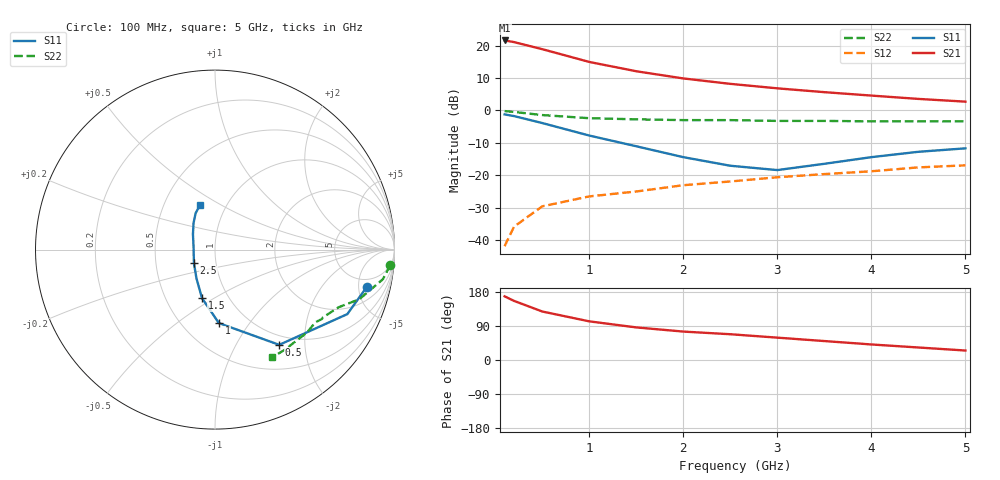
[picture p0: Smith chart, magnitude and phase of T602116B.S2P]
!AT-60211
!S-PARAMETERS at Vce=6V  Ic=5mA.  LAST UPDATED 07-21-92
# ghz s ma r 50
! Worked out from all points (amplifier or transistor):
!   12 points, 100 MHz to 5 GHz, reference 50 ohm
!   highest |S21| = 21.6 dB at 100 MHz (marker M1)
!   |S21| within 3 dB of that: start of sweep to 539.3 MHz
!   unconditionally stable (mu >= 1): 1.411 GHz to end of sweep
!   at 500 MHz: K = 0.50, MSG = 24.3 dB, |S12| = -29.6 dB
!   at 2.5 GHz: K = 1.22, MAG = 12.3 dB, |S12| = -21.9 dB
!   at 5 GHz: K = 1.23, MAG = 6.9 dB, |S12| = -17.0 dB
!   S11 on the Smith chart (normalised r, x): 100 MHz: 3.54, -6.14; 500 MHz: 0.85, -1.53; 1 GHz: 0.74, -0.73; 1.5 GHz: 0.75, -0.44; 2.5 GHz: 0.78, -0.12; 5 GHz: 0.75, +0.40
0.1  0.87 -14.0  12.09 168.0  0.008 80.0  0.98 -5.0
0.2  0.82 -26.0  11.41 156.0  0.016 80.0  0.95 -10.0
0.5  0.64 -56.0  8.87 128.0  0.033 59.0  0.85 -19.0
1  0.41 -87.0  5.63 102.0  0.047 54.0  0.76 -25.0
1.5  0.28 -105.0  4.04 86.0  0.056 54.0  0.73 -29.0
2  0.19 -123.0  3.13 75.0  0.07 56.0  0.71 -32.0
2.5  0.14 -147.0  2.58 68.0  0.08 60.0  0.71 -33.0
3  0.12 174.0  2.2 59.0  0.093 58.0  0.69 -36.0
3.5  0.15 145.0  1.92 50.0  0.104 58.0  0.69 -42.0
4  0.19 129.0  1.7 41.0  0.115 56.0  0.68 -49.0
4.5  0.23 118.0  1.51 33.0  0.132 53.0  0.68 -55.0
5  0.26 109.0  1.37 25.0  0.142 53.0  0.68 -62.0
